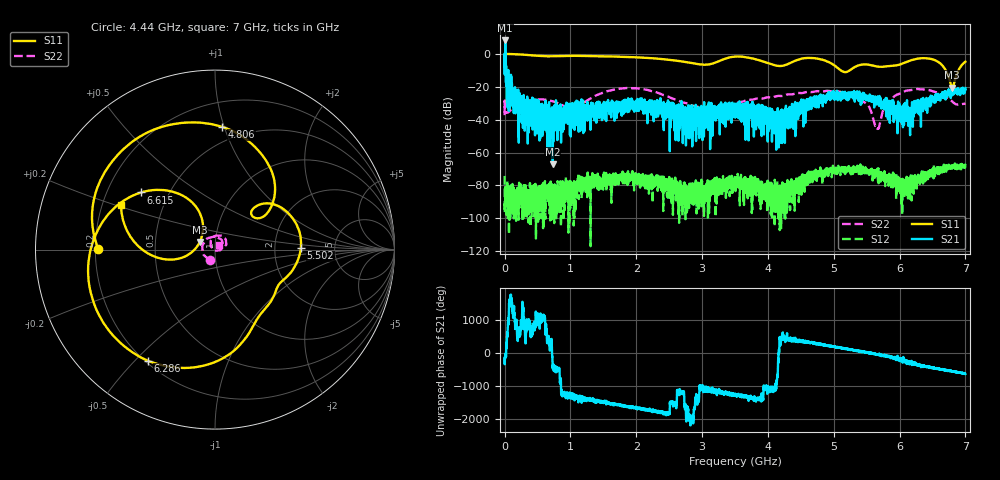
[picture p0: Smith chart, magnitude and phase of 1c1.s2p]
!Keysight Technologies,N5232A,MY52221221,A.10.65.11
!Date: Wednesday, October 16, 2024 12:00:09
!Correction: S11(Full 2 Port(1,4))
!S41(Full 2 Port(1,4))
!S14(Full 2 Port(1,4))
!S44(Full 2 Port(1,4))
!S2P File: Measurements: S11, S41, S14, S44:
# Hz S  RI  R 50
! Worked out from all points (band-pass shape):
!   4001 points, 300 kHz to 7 GHz, reference 50 ohm
!   highest |S21| = 8.19 dB at 10.8 MHz (marker M1); lowest = -67.0 dB at 731.8 MHz (marker M2)
!   |S21| within 3 dB of the highest: 9.116 MHz to 11.12 MHz (1.999 MHz wide, 19.8 % of centre)
!   lowest |S11| = -20.4 dB at 6.801 GHz (marker M3), VSWR 1.21, Z = 42 + j3.56 ohm
!   |S11| at or under -10 dB: 5.108 GHz to 5.243 GHz (134.9 MHz wide, 2.61 % of centre); 6.703 GHz to 6.894 GHz (191.5 MHz wide, 2.82 % of centre)
!   |S22| runs from -45.6 to -20.7 dB; largest |S21 - S12| = 2.6
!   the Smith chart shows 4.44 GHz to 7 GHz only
!   S11 on the Smith chart (normalised r, x): 4.44 GHz: 0.21, +0.00; 4.806 GHz: 0.38, +0.99; 5.502 GHz: 2.83, +0.06; 6.286 GHz: 0.21, -0.54; 6.615 GHz: 0.35, +0.30; 7 GHz: 0.28, +0.21
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300000  -0.9942 -0.0119  -0.8581 -0.4993  -0.000123 -0.000152  -0.0116 -0.00742
1.079955e7  -0.9989 0.0373  -0.236 -2.556  -1.63e-05 2.66e-05  -0.0167 0.00217
5.979745e7  -0.9736 0.1997  -0.0616 -0.0871  -4.43e-06 2.36e-05  -0.0131 0.0109
1.910418e8  -0.7816 0.5792  -0.0268 0.0248  3.26e-06 1.81e-05  0.00177 0.0261
7.317686e8  0.5017 0.6836  0.000441 6.06e-05  -3.74e-05 -0.000106  0.0243 -0.027
1.1675e9  0.8251 -0.2846  0.00239 0.0323  0.000123 -7.9e-05  -0.0195 0.0214
1.669728e9  -0.1813 -0.8132  -0.00525 -0.00769  -9.25e-06 0.000192  0.0833 0.00292
2.014464e9  -0.746 -0.248  -0.00769 0.022  0.000123 -0.000111  0.0345 -0.0829
2.3347e9  -0.5696 0.4314  0.0159 0.0212  -6.44e-05 3.11e-05  -0.0485 -0.0441
3.228912e9  0.5103 0.2595  0.00418 -0.0222  6.68e-05 -0.000167  -0.00228 -0.0181
3.50015e9  0.7061 -0.4323  -0.0182 -0.00315  -0.000157 -1.37e-05  -0.0277 0.0122
3.872884e9  -0.2821 -0.5723  0.00583 0.00817  6.59e-05 2.53e-05  0.0282 0.034
4.43986e9  -0.6511 0.00568  0.0133 0.0124  7.1e-05 -9.41e-05  -0.0288 -0.0581
4.66735e9  -0.3951 0.643  0.0314 -0.0229  -0.000189 5.88e-05  -0.0688 -0.00514
4.805594e9  0.041 0.6834  0.0085 -0.0423  -0.000108 0.000155  -0.0625 0.0358
5.502064e9  0.4779 0.00811  0.0454 0.0166  -0.000289 8.75e-05  0.0298 -0.00348
5.661307e9  0.3755 -0.1738  0.0346 -0.0248  2.03e-06 0.000222  -0.00214 -0.00497
5.83455e9  0.3085 -0.2924  -0.00423 -0.0218  0.000197 5.64e-05  -0.0244 0.0234
6.286031e9  -0.3753 -0.6184  0.0305 -0.00196  6.27e-05 0.000141  0.0401 0.0755
6.615016e9  -0.4128 0.3182  -0.0256 -0.0412  -0.000154 -0.000236  0.0575 0.0219
6.800509e9  -0.0853 0.042  -0.0803 -0.00141  -0.000258 0.000246  0.0346 0.00953
7e9  -0.5233 0.2488  -0.0139 0.0905  0.000341 0.000233  0.0208 0.0229
